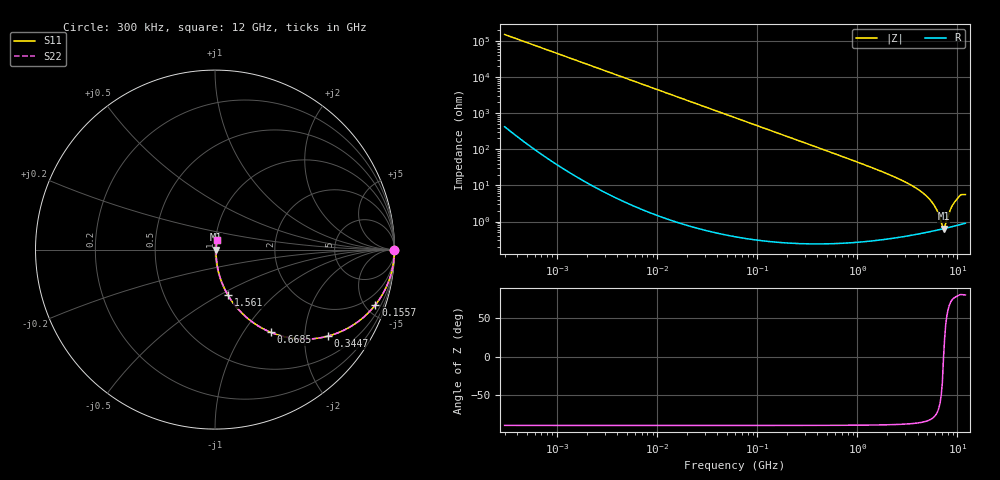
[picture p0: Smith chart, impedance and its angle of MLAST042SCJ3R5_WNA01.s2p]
! MLAST042SCJ3R5_WNA01  S-PARAMETER MODEL  ( General Type )
! Model Generated by TAIYO YUDEN Corporation (http://www.ty-top.com)
! Version 1.0
! TAIYO YUDEN Control No. 150820
! Copyright(c) 2015 TAIYO YUDEN CO.,LTD. All Rights Reserved.
! Product Description (link to TY-COMPAS)
! https://ds.yuden.co.jp/TYCOMPAS/or/detail?pn=MLAST042SCJ3R5BWNA01&u=M
! Products Name : Multilayer Ceramic Capacitors
! Characteristics :
!  Capacitance : 3.5 pF , Rated Voltage : 25V , TCC : CJ / C0J
!  Case Size : 0.4 x 0.2 / 0.016 x 0.008 [mm/inch] , Thickness : 0.2 / 0.008 [mm/inch]
!  (Conditions: Temperature = 25 degC , DC Bias Current/Voltage = 0A / 0V)
! External Node Assignments :
!  1  o---| |---o  2
! GND o---------o GND
! Frequency Range : 0.3MHz  -  12000MHz  [ 401 STEP ]
# MHz S RI R 50
! Freq[MHz].  S11 Real  S11 Imag  S21 Real  S21 Imag  S12 Real  S12 Imag  S22 Real  S22 Imag
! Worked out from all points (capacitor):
!   401 points, 300 kHz to 12 GHz, reference 50 ohm
!   read as one part in series: C = 3.53 pF near 316.3 kHz
!   lowest |Z| = 635 mohm at 7.254 GHz (marker M1)
!   series resonance near 7.266 GHz, so ESL is about 140 pH
!   S11 on the Smith chart (normalised r, x): 300 kHz: open; 155.7 MHz: 1.01, -5.80; 344.7 MHz: 1.00, -2.61; 668.5 MHz: 1.00, -1.34; 1.561 GHz: 1.01, -0.55; 12 GHz: 1.02, +0.11
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0.3  1 -0.000665  2.3e-06 0.000665  2.3e-06 0.000665  1 -0.000665
1.769972  1 -0.00392  1.76e-05 0.00392  1.76e-05 0.00392  1 -0.00392
10.44266  0.9995 -0.0231  0.000542 0.0231  0.000542 0.0231  0.9995 -0.0231
60  0.9826 -0.1306  0.0174 0.1306  0.0174 0.1306  0.9826 -0.1306
155.7172  0.8934 -0.3082  0.1066 0.3082  0.1066 0.3082  0.8934 -0.3082
344.7396  0.6304 -0.4818  0.3696 0.4818  0.3696 0.4818  0.6304 -0.4818
353.9943  0.6179 -0.485  0.3821 0.485  0.3821 0.485  0.6179 -0.485
668.5285  0.3102 -0.4607  0.6898 0.4607  0.6898 0.4607  0.3102 -0.4607
1021.415  0.1596 -0.3632  0.8404 0.3632  0.8404 0.3632  0.1596 -0.3632
1560.575  0.0732 -0.2551  0.9268 0.2551  0.9268 0.2551  0.0732 -0.2551
2088.533  0.0409 -0.1898  0.9591 0.1898  0.9591 0.1898  0.0409 -0.1898
3454.93  0.0142 -0.0996  0.9858 0.0996  0.9858 0.0996  0.0142 -0.0996
4875.354  0.00757 -0.0508  0.9924 0.0508  0.9924 0.0508  0.00757 -0.0508
5868.704  0.00627 -0.027  0.9937 0.027  0.9937 0.027  0.00627 -0.027
6354.153  0.0061 -0.0171  0.9939 0.0171  0.9939 0.0171  0.0061 -0.0171
6879.757  0.00616 -0.0074  0.9938 0.0074  0.9938 0.0074  0.00616 -0.0074
7254.098  0.00631 -0.000184  0.9937 0.000184  0.9937 0.000184  0.00631 -0.000184
7648.807  0.00657 0.00613  0.9934 -0.00613  0.9934 -0.00613  0.00657 0.00613
8503.825  0.0074 0.02  0.9926 -0.02  0.9926 -0.02  0.0074 0.02
9454.42  0.00872 0.0345  0.9913 -0.0345  0.9913 -0.0345  0.00872 0.0345
10793.46  0.0111 0.0535  0.9889 -0.0535  0.9889 -0.0535  0.0111 0.0535
12000  0.0119 0.0541  0.9881 -0.0541  0.9881 -0.0541  0.0119 0.0541
